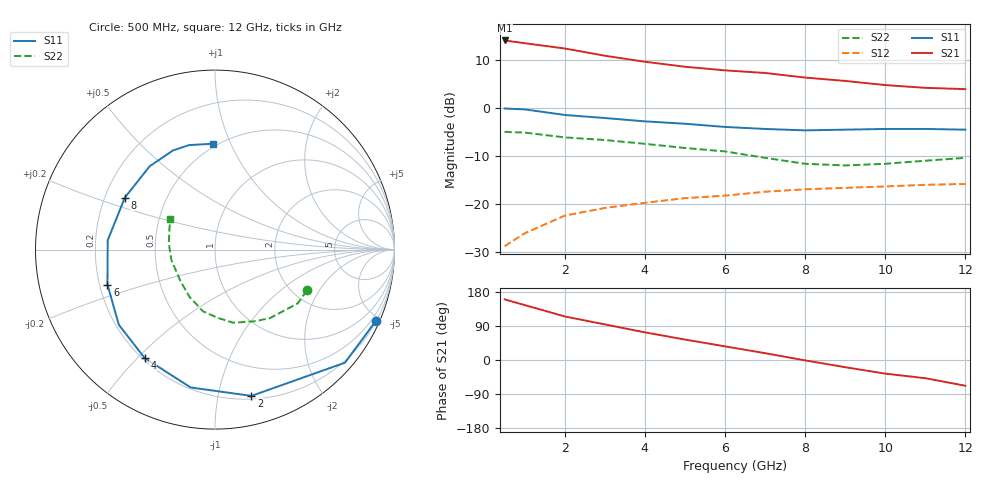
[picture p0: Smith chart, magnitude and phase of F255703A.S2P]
!ATF-25570
!S-PARAMETERS at Vds=3V  Id=20mA.  LAST UPDATED 07-22-92
# ghz s ma r 50
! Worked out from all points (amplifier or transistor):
!   13 points, 500 MHz to 12 GHz, reference 50 ohm
!   highest |S21| = 14.0 dB at 500 MHz (marker M1)
!   |S21| within 3 dB of that: start of sweep to 2.879 GHz
!   unconditionally stable (mu >= 1): 7.204 GHz to end of sweep
!   at 2 GHz: K = 0.40, MSG = 17.4 dB, |S12| = -22.5 dB
!   at 6 GHz: K = 0.93, MSG = 13.1 dB, |S12| = -18.3 dB
!   at 12 GHz: K = 1.14, MAG = 7.6 dB, |S12| = -15.9 dB
!   S11 on the Smith chart (normalised r, x): 500 MHz: 0.23, -4.69; 2 GHz: 0.23, -1.25; 4 GHz: 0.21, -0.52; 6 GHz: 0.23, -0.15; 8 GHz: 0.28, +0.25; 12 GHz: 0.48, +0.86
0.5  0.98 -24.0  5.02 160.0  0.036 71.0  0.56 -24.0
1  0.96 -41.0  4.7 145.0  0.049 62.0  0.55 -33.0
2  0.84 -76.0  4.14 115.0  0.075 44.0  0.49 -51.0
3  0.78 -100.0  3.48 94.0  0.09 33.0  0.46 -60.0
4  0.72 -123.0  3.01 73.0  0.102 20.0  0.42 -76.0
5  0.68 -142.0  2.67 54.0  0.114 9.0  0.38 -88.0
6  0.63 -162.0  2.45 36.0  0.121 0.0  0.35 -101.0
7  0.6 175.0  2.3 18.0  0.133 -7.0  0.3 -118.0
8  0.58 150.0  2.06 -1.0  0.141 -16.0  0.26 -138.0
9  0.59 128.0  1.9 -19.0  0.146 -28.0  0.25 -167.0
10  0.6 113.0  1.72 -36.0  0.151 -35.0  0.26 172.0
11  0.6 104.0  1.61 -48.0  0.157 -40.0  0.28 155.0
12  0.59 91.0  1.56 -68.0  0.16 -44.0  0.3 146.0
